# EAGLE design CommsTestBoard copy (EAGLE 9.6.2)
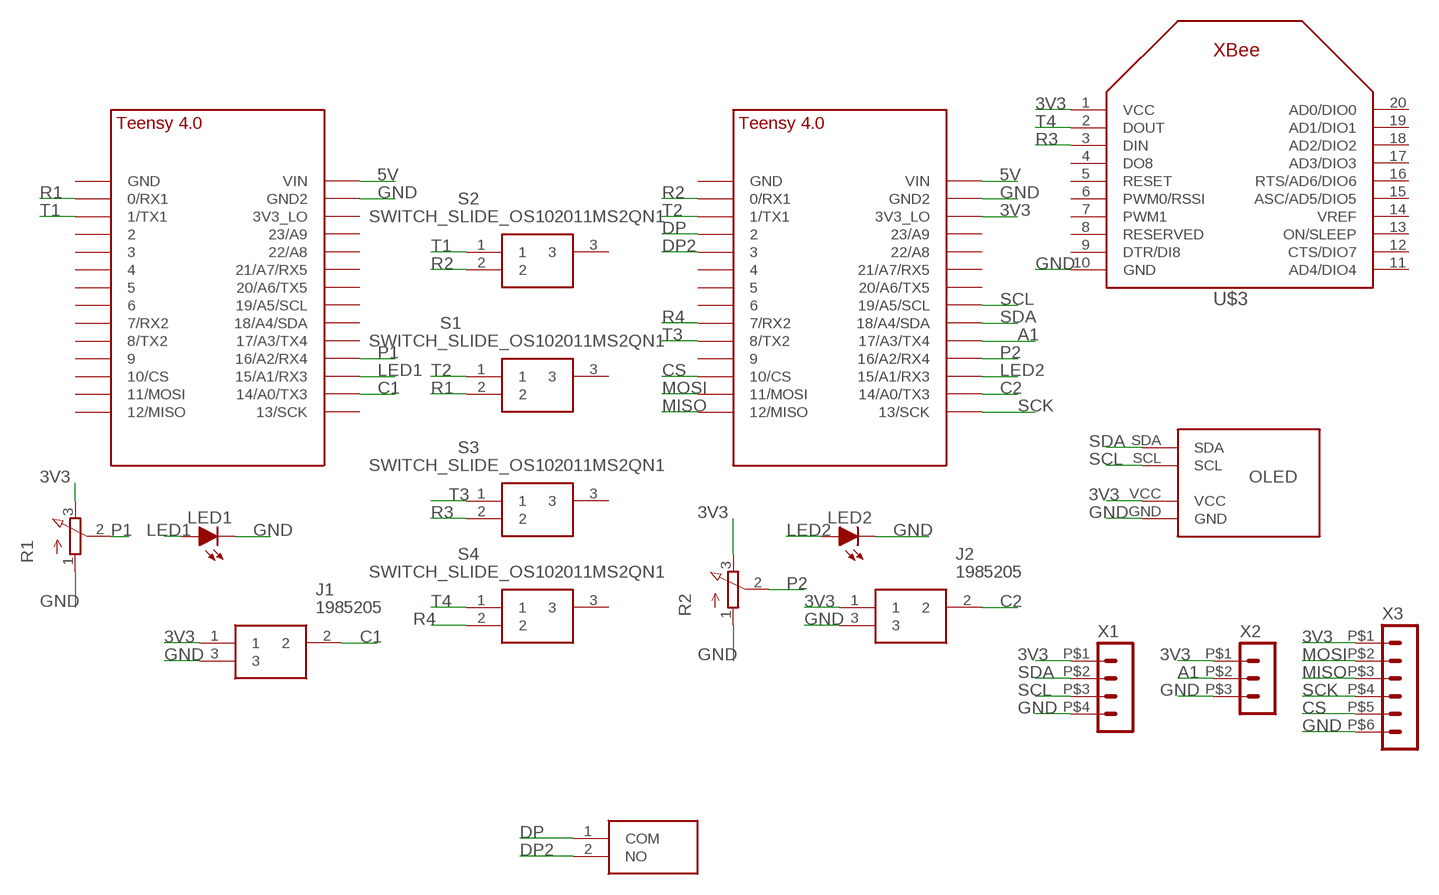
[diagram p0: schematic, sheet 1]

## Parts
J1  1985205  [1985205]
J2  1985205  [1985205]
LED1  LED-5MM  [LED-5MM]
LED2  LED-5MM  [LED-5MM]
R1  POTENTIOMETER  [3RP/1610N]
R2  POTENTIOMETER  [3RP/1610N]
S1  SWITCH_SLIDE_OS102011MS2QN1  [OS102011MA1QN1]
S2  SWITCH_SLIDE_OS102011MS2QN1  [OS102011MA1QN1]
S3  SWITCH_SLIDE_OS102011MS2QN1  [OS102011MA1QN1]
S4  SWITCH_SLIDE_OS102011MS2QN1  [OS102011MA1QN1]
S5  PTS636_SL50_LFS  [PTS636SL50LFS]
U$1  TEENSY_4.0_SIMPLE  [TEENSY_4.0_SIMPLE]
U$2  TEENSY_4.0_SIMPLE  [TEENSY_4.0_SIMPLE]
U$3  XBEE  [XBEE]
U$4  OLED_SSD1306  [OLED_SSD1306]
X1  HEADER_POS4_43045-0401  [43045-0400]
X2  HEADER_POS3_43650-0300  [43650-0300]
X3  HEADER_POS6_43045-0600  [43045-0600]

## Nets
3V3: J1.1 J2.1 R1.3(E) R2.3(E) U$2.3V3_LO U$3.1(VCC) U$4.VCC X1.P$1 X2.P$1 X3.P$1
5V: U$1.VIN U$2.VIN
A1: U$2.17/A3(17/A3/TX4) X2.P$2
C1: J1.2 U$1.14/A0(14/A0/TX3)
C2: J2.2 U$2.14/A0(14/A0/TX3)
CS: U$2.10/CS X3.P$5
DP: S5.1(COM) U$2.2
DP2: S5.2(NO) U$2.3/CANTX
GND: J1.3 J2.3 LED1.K(C) LED2.K(C) R1.1(A) R2.1(A) U$1.GND2 U$2.GND2 U$3.10(GND) U$4.GND X1.P$4 X2.P$3 X3.P$6
LED1: LED1.A U$1.15/A1(15/A1/RX3)
LED2: LED2.A U$2.15/A1(15/A1/RX3)
MISO: U$2.12/MISO X3.P$3
MOSI: U$2.11/MOSI X3.P$2
P1: R1.2(S) U$1.16/A2(16/A2/RX4)
P2: R2.2(S) U$2.16/A2(16/A2/RX4)
R1: S1.2 U$1.0/RX(0/RX1)
R2: S2.2 U$2.0/RX(0/RX1)
R3: S3.2 U$3.3(DIN)
R4: S4.2 U$2.7(7/RX2)
SCK: U$2.13/SCK X3.P$4
SCL: U$2.19/A5/SCL U$4.SCL X1.P$3
SDA: U$2.18/A4/SDA U$4.SDA X1.P$2
T1: S2.1 U$1.1/TX(1/TX1)
T2: S1.1 U$2.1/TX(1/TX1)
T3: S3.1 U$2.8(8/TX2)
T4: S4.1 U$3.2(DOUT)
Unconnected: S1.3 S2.3 S3.3 S4.3 U$1.2 U$1.3/CANTX U$1.3V3_LO U$1.4/CANRX U$1.5 U$1.6 U$1.7(7/RX2) U$1.8(8/TX2) U$1.9/CS U$1.10/CS U$1.11/MOSI U$1.12/MISO U$1.13/SCK U$1.17/A3(17/A3/TX4) U$1.18/A4/SDA U$1.19/A5/SCL U$1.20/A6(20/A6/TX5) U$1.21/A7(21/A7/RX5) U$1.22/A8 U$1.23/A9 U$1.GND U$2.4/CANRX U$2.5 U$2.6 U$2.9/CS U$2.20/A6(20/A6/TX5) U$2.21/A7(21/A7/RX5) U$2.22/A8 U$2.23/A9 U$2.GND U$3.4(DO8) U$3.5(RESET) U$3.6(PWM0/RSSI) U$3.7(PWM1) U$3.8(RESERVED) U$3.9(DTR/DI8) U$3.11(AD4/DIO4) U$3.12(CTS/DIO7) U$3.13(ON/SLEEP) U$3.14(VREF) U$3.15(ASC/AD5/DIO5) U$3.16(RTS/AD6/DIO6) U$3.17(AD3/DIO3) U$3.18(AD2/DIO2) U$3.19(AD1/DIO1) U$3.20(AD0/DIO0)

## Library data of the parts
J1 J2 = GTOR - Connectors:1985205: Fixed Terminal Blocks PTSA 1.5/3-3.5-Z Source: Datasheet; ARROW_PART_NUMBER: 1985205; ARROW_PRICE-STOCK: https://www.arrow.com/en/products/1985205/phoenix-contact; DESCRIPTION: Fixed Terminal Blocks PTSA 1.5/3-3.5-Z; HEIGHT: 13mm; MANUFACTURER_NAME: Phoenix Contact; MANUFACTURER_PART_NUMBER: 1985205; MOUSER_PART_NUMBER: 651-1985205; MOUSER_PRICE-STOCK: https://www.mouser.co.uk/ProductDetail/Phoenix-Contact/1985205?qs=JcjeNNoqGSNoFnucoMlHJQ%3D%3D
LED1 LED2 = GTOR - Passive Components:LED: Light Emitting Diode (LED)
R1 R2 = GTOR - Passive Components:POTENTIOMETER: 16mm Potentiometer one level Source: http://www.alphapotentiometers.net/html/16mm_pot_2.html
S1-S4 = GTOR - Active Components:SWITCH_SLIDE_OS102011MS2QN1: Switch Slide Miniature SPDT 0.1A 12VDC Through Hole Slide Switch SPDT On-On 0.1 A@ 12 V dc Slide Source: Datasheet; ARROW_PART_NUMBER: OS102011MS2QN1; ARROW_PRICE-STOCK: https://www.arrow.com/en/products/os102011ms2qn1/ck; DESCRIPTION: Switch Slide Miniature SPDT 0.1A 12VDC Through Hole Slide Switch SPDT On-On 0.1 A@ 12 V dc Slide; HEIGHT: mm; MANUFACTURER_NAME: C & K COMPONENTS; MANUFACTURER_PART_NUMBER: OS102011MS2QN1; MOUSER_PART_NUMBER: 611-OS102011MS2QN1; MOUSER_PRICE-STOCK: https://www.mouser.co.uk/ProductDetail/CK/OS102011MS2QN1?qs=WtljUlYws5RvQ1hEv876nQ%3D%3D
S5 = GTOR - Active Components:PTS636_SL50_LFS: Tactile Switches Tact 50mA 12VDC, 6.0x3.5, 5.0mm H, 130gf, THT leads, Black Actuator; ARROW_PART_NUMBER: PTS636 SL50 LFS; ARROW_PRICE-STOCK: https://www.arrow.com/en/products/pts636-sl50-lfs/ck; DESCRIPTION: Tactile Switches Tact 50mA 12VDC, 6.0x3.5, 5.0mm H, 130gf, THT leads, Black Actuator; HEIGHT: 5.2mm; MANUFACTURER_NAME: C & K COMPONENTS; MANUFACTURER_PART_NUMBER: PTS636 SL50 LFS; MOUSER_PART_NUMBER: 611-PTS636SL50LFS; MOUSER_PRICE-STOCK: https://www.mouser.co.uk/ProductDetail/CK/PTS636-SL50-LFS?qs=vLWxofP3U2xbACAJDYC1Hw%3D%3D
U$1 U$2 = GTOR - Microcontroller:TEENSY_4.0_SIMPLE
U$3 = GTOR - Microcontroller:XBEE: Source: Adafruit
U$4 = GTOR - Breakout Boards:OLED_SSD1306
X1 = GTOR - Microfit Connector:HEADER_POS4_?: Molex - Micro-Fit 3.0 Series connector, 3.00mm (0.118") pitch header, 4 positions.
X2 = GTOR - Microfit Connector:HEADER_POS3_?: Molex - Micro-Fit 3.0 Series connector, 3.00mm (0.118") pitch header, 3 positions.
X3 = GTOR - Microfit Connector:HEADER_POS6_?: Molex - Micro-Fit 3.0 Series connector, 3.00mm (0.118") pitch header, 6 positions.

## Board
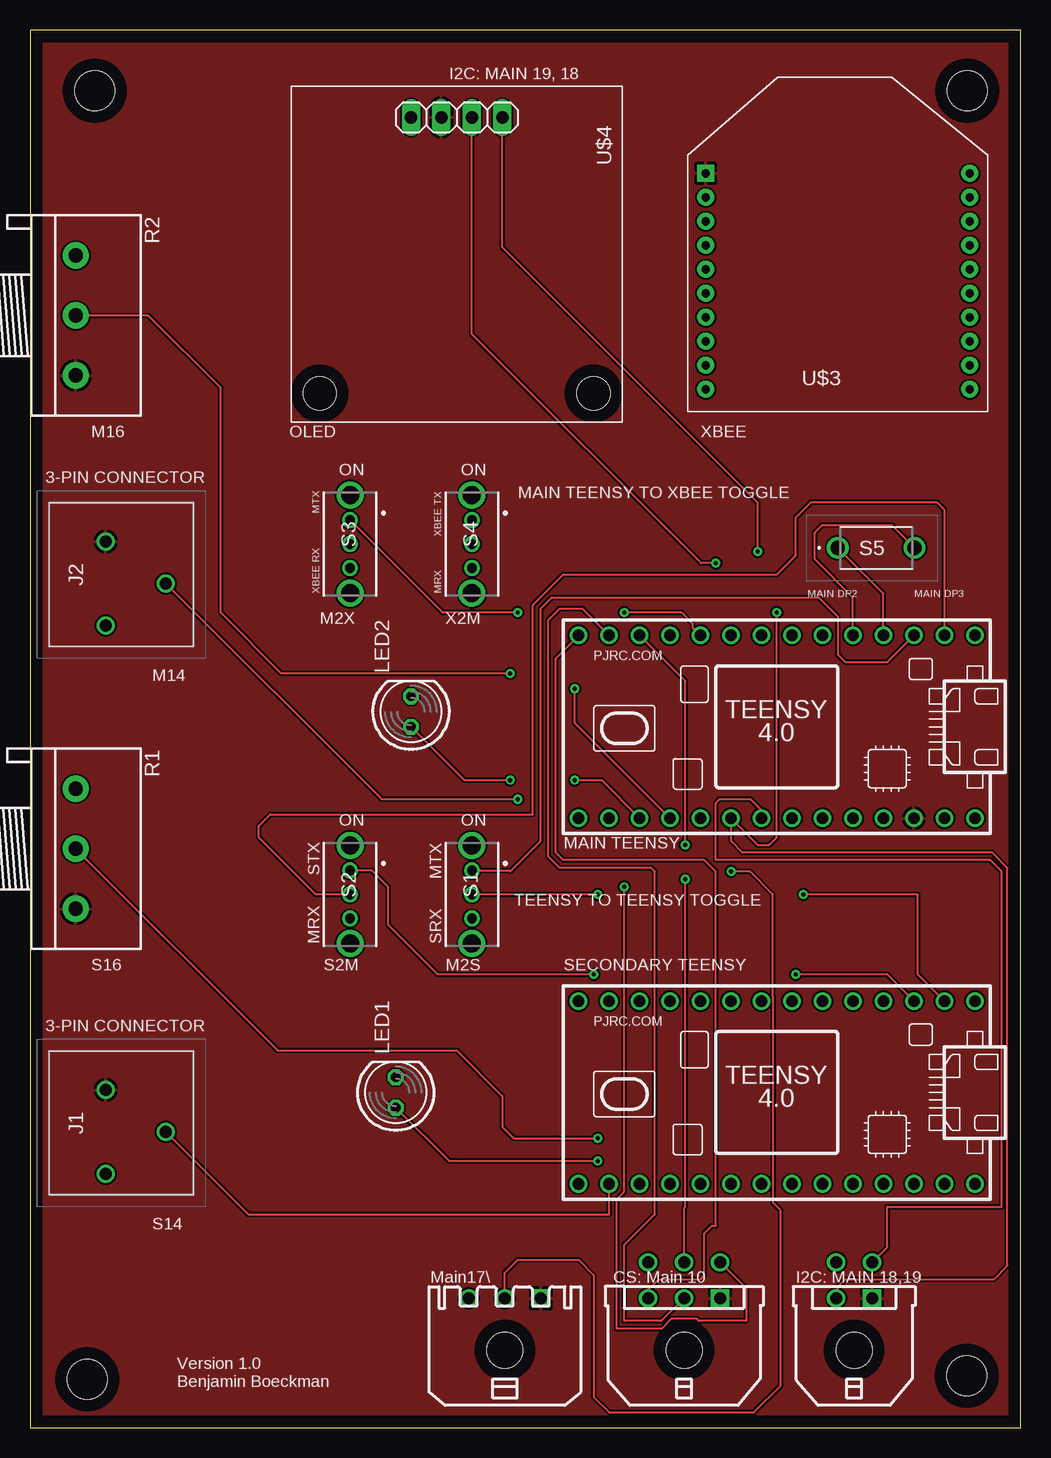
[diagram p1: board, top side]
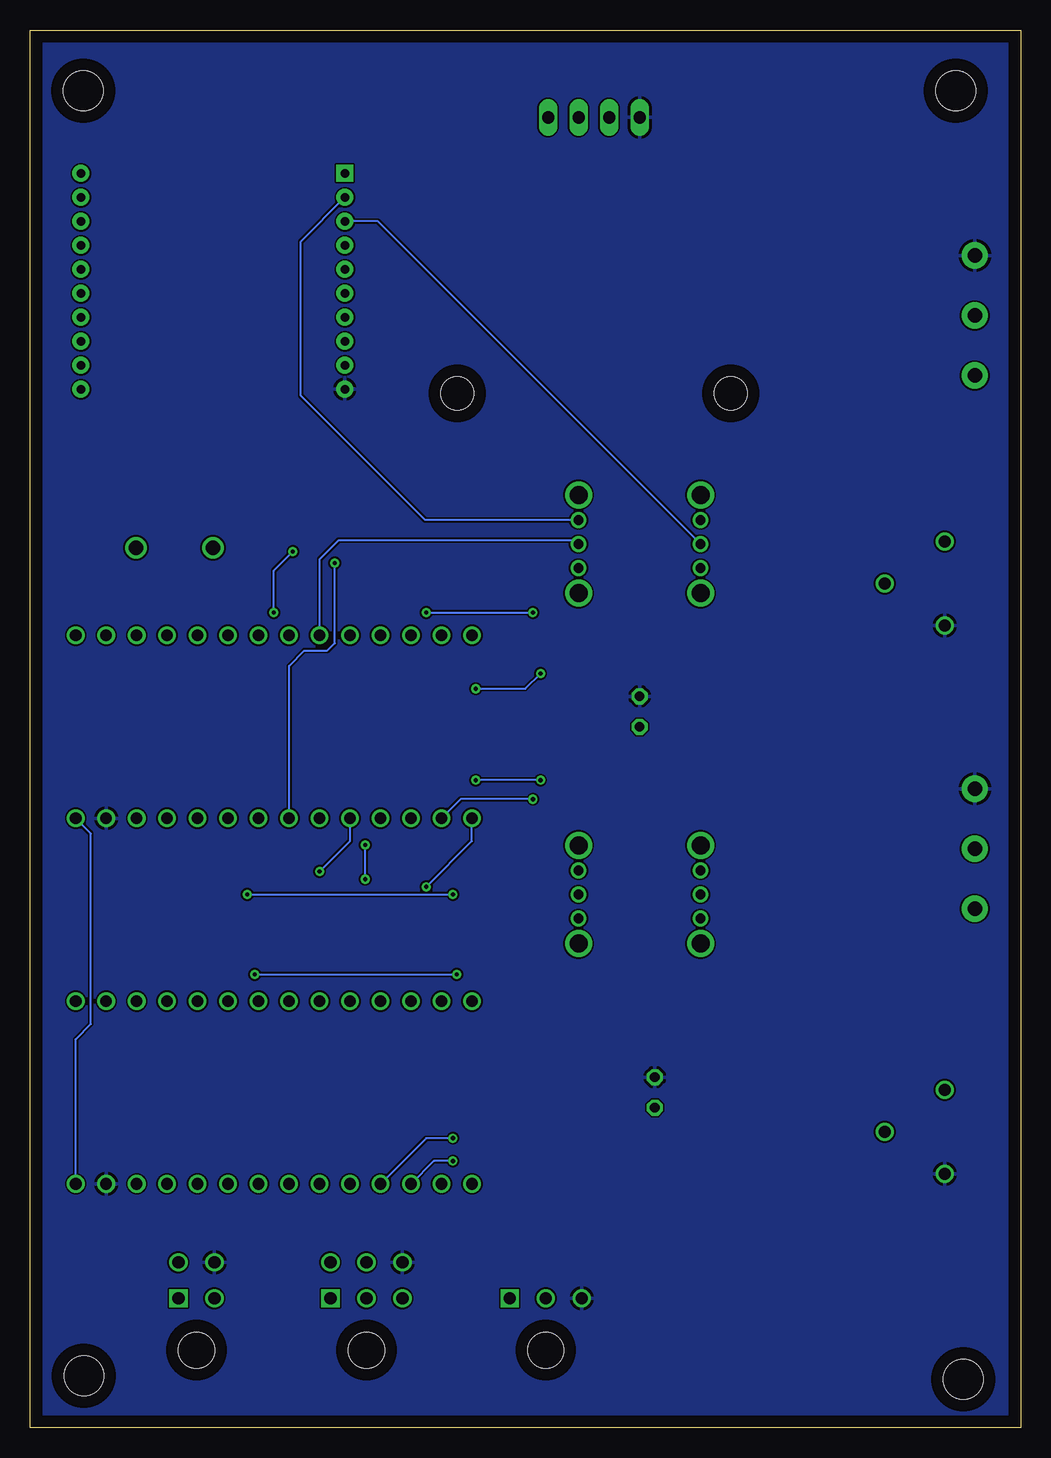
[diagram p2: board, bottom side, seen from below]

Size 82.55 x 116.51 mm. Coordinates in mm from the lower left corner, seen from the top.
Outline: 82.55,0 82.55,116.51 0,116.51 0,0 82.55,0
Copper layers (1*16): Top 0.035mm / dielectric 1.5mm / Bottom 0.035mm
Design rules "default": minimum track width 6mil, minimum drill 0.35mm, track to track 6mil, track to pad 6mil, pad to pad 6mil, via to via 6mil, smd to smd 6mil, copper to edge 40mil, drill to drill 6mil, minimum pad ring 10mil, minimum via ring 8mil, stop-mask expansion 4mil, vias tented up to drill 0mil, thermal gap 10mil
Holes 3.3 mm at 4.78,4.03 5.4,111.44 78.1,111.44 78.05,4.32
Holes 2.75 mm at 24.15,86.21 46.95,86.21

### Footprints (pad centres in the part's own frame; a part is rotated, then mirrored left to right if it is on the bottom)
1985205 = drill 1 pad 1.5: 1 -2.75,-1.3; 2 0.75,3.7; 3 4.25,-1.3
LED-5MM = drill 0.813 octagon: A -1.27,0; K 1.27,0
3RP/1610N = drill 1.2 pad 2.184: 1 -5,0; 2 0,0; 3 5,0
OS102011MA1QN1 = drill 0.8 pad 1.3: 1 -2,0; 2 0,0; 3 2,0 | drill 1.5 pad 2.25: 4 -4.1,0; 5 4.1,0
PTS636SL50LFS = drill 1.2 pad 1.8: 1 0,0; 2 6.4,0
TEENSY_4.0_SIMPLE = drill 0.965: 0/RX -13.97,-7.62; 1/TX -11.43,-7.62; 2 -8.89,-7.62; 3/CANTX -6.35,-7.62; 3V3_LO -11.43,7.62; 4/CANRX -3.81,-7.62; 5 -1.27,-7.62; 6 1.27,-7.62; 7 3.81,-7.62; 8 6.35,-7.62; 9/CS 8.89,-7.62; 10/CS 11.43,-7.62; 11/MOSI 13.97,-7.62; 12/MISO 16.51,-7.62; 13/SCK 16.51,7.62; 14/A0 13.97,7.62; 15/A1 11.43,7.62; 16/A2 8.89,7.62; 17/A3 6.35,7.62; 18/A4/SDA 3.81,7.62; 19/A5/SCL 1.27,7.62; 20/A6 -1.27,7.62; 21/A7 -3.81,7.62; 22/A8 -6.35,7.62; 23/A9 -8.89,7.62; GND -16.51,-7.62; GND2 -13.97,7.62; VIN -16.51,7.62
XBEE = drill 0.7 pad 1.422 square: 1 -11,5.5 | drill 0.7 pad 1.422: 2 -11,3.5; 3 -11,1.5; 4 -11,-0.5; 5 -11,-2.5; 6 -11,-4.5; 7 -11,-6.5; 8 -11,-8.5; 9 -11,-10.5; 10 -11,-12.5; 11 11,-12.5; 12 11,-10.5; 13 11,-8.5; 14 11,-6.5; 15 11,-4.5; 16 11,-2.5; 17 11,-0.5; 18 11,1.5; 19 11,3.5; 20 11,5.5
OLED_SSD1306 = drill 1.016 long: GND 0,-3.81; SCL 0,1.27; SDA 0,3.81; VCC 0,-1.27
43045-0400 = drill 1.02 square: P$1 1.5,4.32 | drill 1.02: P$2 -1.5,4.32; P$3 1.5,7.32; P$4 -1.5,7.32 | hole 3: 0,0
43650-0300 = drill 1.02 square: P$1 3,4.32 | drill 1.02: P$2 0,4.32; P$3 -3,4.32 | hole 3: 0,0
43045-0600 = drill 1.02 square: P$1 3,4.32 | drill 1.02: P$2 0,4.32; P$3 -3,4.32; P$4 3,7.32; P$5 0,7.32; P$6 -3,7.32 | hole 3: 0,0

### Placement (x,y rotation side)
J1  7.62,25.4 270 top
J2  7.62,71.12 270 top
LED1  30.48,27.94 90 top
LED2  31.75,59.69 90 top
R1  3.81,48.26 270 top
R2  3.81,92.71 270 top
S1  36.83,44.45 270 top
S2  26.67,44.45 270 top
S3  26.67,73.66 270 top
S4  36.83,73.66 270 top
S5  67.31,73.34 0 top
U$1  62.23,27.94 180 top
U$2  62.23,58.42 180 top
U$3  67.31,99.06 0 top
U$4  35.56,109.22 270 top
X1  68.68,6.46 0 top
X2  39.57,6.46 0 top
X3  54.51,6.46 0 top

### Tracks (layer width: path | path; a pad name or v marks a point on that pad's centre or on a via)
3V3
  pour Top: 0,116.52 82.55,116.52 82.55,0 0,0
5V
  Bottom 0.152: U$1.VIN 78.74,32.39 77.47,33.66 77.47,49.53 U$2.VIN
A1  (via drill 0.35)
  Top 0.152: v58.42,46.36 60.01,46.36 61.91,44.45 61.91,35.97 61.93,35.96 61.93,18.72 62.55,18.1 62.55,3.49 60.33,1.27 48.26,1.27 46.99,2.54 46.99,12.7 45.72,13.97 40.64,13.97 39.57,12.9 X2.P$2
  Bottom 0.152: v58.42,46.36 55.88,48.89 U$2.17/A3
C1
  Top 0.152: J1.2 18.19,17.78 48.26,17.78 U$1.14/A0
C2  (via drill 0.35)
  Top 0.152: J2.2 29.3,52.39 v40.64,52.39
  Bottom 0.152: v40.64,52.39 46.67,52.39 U$2.14/A0
CS  (via drill 0.35)
  Top 0.152: v54.61,48.58 54.61,62.23 U$2.10/CS | v54.61,45.72 54.61,18.42 54.51,18.32 X3.P$5
  Bottom 0.152: v54.61,45.72 v54.61,48.58
DP
  Top 0.152: U$2.2 71.12,69.53 S5.1
DP2
  Top 0.152: U$2.3/CANTX 68.58,69.22 65.41,72.39 65.41,74.61 66.04,75.25 71.8,75.25 S5.2
GND
  pour Bottom: 0,0 82.55,0 82.55,116.84 0,116.84
LED1  (via drill 0.35)
  Top 0.152: LED1.A 34.92,22.23 v47.31,22.23
  Bottom 0.152: v47.31,22.23 48.9,22.23 U$1.15/A1
LED2  (via drill 0.35)
  Top 0.152: LED2.A 36.2,53.98 v40.01,53.98 | v45.4,53.98 47.62,53.98 U$2.15/A1
  Bottom 0.152: v40.01,53.98 v45.4,53.98
MISO
  Top 0.152: U$2.12/MISO 43.82,64.14 43.82,47.94 44.45,47.31 56.2,47.31 57.15,46.36 57.15,16.83 56.83,16.83 56.2,16.19 56.2,12.7 55.88,12.38 52.39,12.38 51.51,11.51 X3.P$3
MOSI
  Top 0.152: U$2.11/MOSI 46.04,68.26 44.13,68.26 43.18,67.31 43.18,47.62 44.13,46.67 51.75,46.67 52.07,46.36 52.07,17.78 49.53,15.24 49.53,8.89 52.62,8.89 X3.P$2
P1  (via drill 0.35)
  Top 0.152: R1.2 20.64,31.43 35.56,31.43 39.37,27.62 39.37,25.08 40.32,24.13 v47.31,24.13
  Bottom 0.152: v47.31,24.13 49.53,24.13 U$1.16/A2
P2  (via drill 0.35)
  Top 0.152: U$2.16/A2 45.4,58.74 v45.4,61.59 | v40.01,62.86 20.95,62.86 15.88,67.95 15.88,86.68 9.84,92.71 R2.2
  Bottom 0.152: v45.4,61.59 41.27,61.59 v40.01,62.86
R1  (via drill 0.35)
  Top 0.152: U$1.0/RX 73.98,37.78 73.98,44.45 v64.45,44.45 | v47.31,44.45 S1.2
  Bottom 0.152: v64.45,44.45 v47.31,44.45
R2
  Top 0.152: S2.2 23.81,44.45 19.05,49.21 19.05,50.17 20,51.12 41.91,51.12 41.91,68.58 44.45,71.12 62.23,71.12 63.82,72.71 63.82,75.88 65.09,77.15 75.56,77.15 76.2,76.52 U$2.0/RX
R3
  Bottom 0.152: S3.2 53.57,100.56 U$3.3
R4
  Bottom 0.152: U$2.7 58.42,72.39 56.83,73.98 37.15,73.98 S4.2
SCK  (via drill 0.35)
  Top 0.152: X3.P$4 59.69,11.6 59.69,8.89 55.75,8.89 55.58,9.05 53.44,9.05 52.64,8.26 48.9,8.26 48.9,19.05 49.52,19.67 49.52,21.01 | 49.52,21.01 49.53,21.03 | 49.52,21.01 49.52,45.07 v49.53,45.09
  Bottom 0.152: v49.53,45.09 45.72,48.89 U$2.13/SCK
SCL  (via drill 0.35)
  Top 0.152: U$2.19/A5/SCL 60.96,51.44 60.01,52.39 57.47,52.39 57.15,52.07 57.15,47.31 80.01,47.31 80.96,46.36 80.96,18.42 71.44,18.42 71.44,15.04 X1.P$3 | U$4.SCL 36.83,91.17 55.93,72.07 v57.15,72.07
  Bottom 0.152: U$2.19/A5/SCL 60.96,63.5 59.69,64.77 57.79,64.77 57.15,65.41 v57.15,72.07
SDA  (via drill 0.35)
  Top 0.152: v62.23,67.95 62.23,49.21 61.59,48.58 60.64,48.58 U$2.18/A4/SDA 58.42,48.89 59.37,47.94 80.19,47.94 81.46,46.67 81.46,13.5 80.34,12.38 67.94,12.38 67.31,11.75 67.31,10.91 X1.P$2 | v60.64,73.03 60.64,77.12 39.37,98.4 U$4.SDA
  Bottom 0.152: v62.23,67.95 62.23,71.44 v60.64,73.03
T1  (via drill 0.35)
  Top 0.152: U$1.1/TX 71.44,37.78 v63.82,37.78 | v46.99,37.78 33.97,37.78 29.84,41.91 29.84,45.09 28.48,46.45 S2.1
  Bottom 0.152: v63.82,37.78 v46.99,37.78
T2
  Top 0.152: S1.1 39.91,46.45 40.01,46.36 42.55,48.89 42.55,68.26 43.5,69.22 65.72,69.22 67.31,67.63 67.31,64.45 67.94,63.82 71.44,63.82 U$2.1/TX
T3  (via drill 0.35)
  Top 0.152: U$2.8 55.25,66.67 55.25,66.99 54.29,67.95 v49.53,67.95 | v40.64,67.95 34.38,67.95 S3.1
  Bottom 0.152: v49.53,67.95 v40.64,67.95
T4
  Bottom 0.152: S4.1 49.62,75.66 60.01,86.04 60.01,98.86 U$3.2

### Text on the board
tPlace: I2C: MAIN 19, 18 | M16 | OLED | XBEE | ON | ON | 3-PIN CONNECTOR | MAIN TEENSY TO XBEE TOGGLE | MTX | XBEE TX | XBEE RX | MRX | MAIN DP2 | MAIN DP3 | M2X | X2M | M14 | ON | ON | MAIN TEENSY | STX | MTX | TEENSY TO TEENSY TOGGLE | MRX | SRX | S16 | S2M | M2S | SECONDARY TEENSY | 3-PIN CONNECTOR | S14 | Main17\ | CS: Main 10 | I2C: MAIN 18,19 | Version 1.0 / Benjamin Boeckman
